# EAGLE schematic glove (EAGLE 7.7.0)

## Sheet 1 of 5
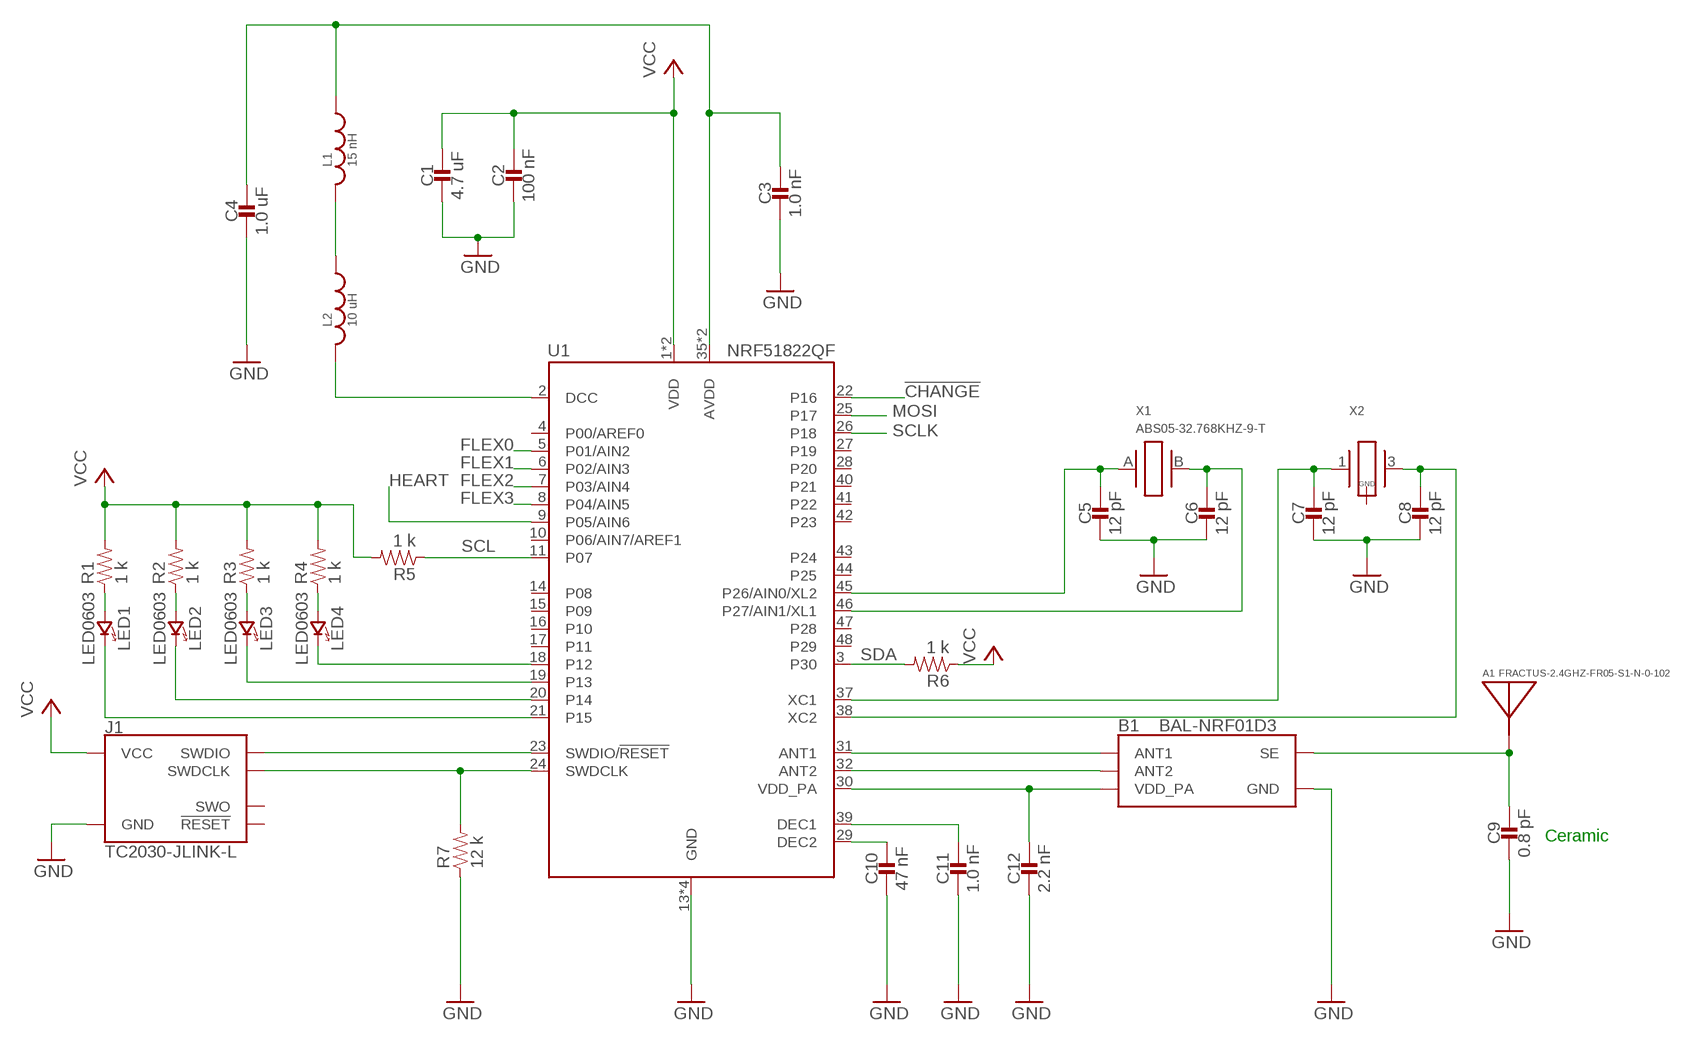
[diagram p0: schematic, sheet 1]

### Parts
A1  FRACTUS-2.4GHZ-FR05-S1-N-0-102  [FRACTUS-ANTENNA-FR05-S1-N-0-102]
B1  BAL-NRF01D3  [BAL-NRF01D3]
C1  4.7 uF  CAPACITOR0603_CAP  [0603_CAP]
C2  100 nF  CAPACITOR0402_CAP  [0402_CAP]
C3  1.0 nF  CAPACITOR0402_CAP  [0402_CAP]
C4  1.0 uF  CAPACITOR0603_CAP  [0603_CAP]
C5  12 pF  CAPACITOR0402_CAP  [0402_CAP]
C6  12 pF  CAPACITOR0402_CAP  [0402_CAP]
C7  12 pF  CAPACITOR0402_CAP  [0402_CAP]
C8  12 pF  CAPACITOR0402_CAP  [0402_CAP]
C9  0.8 pF  CAPACITOR0402_CAP  [0402_CAP]
C10  47 nF  CAPACITOR0402_CAP  [0402_CAP]
C11  1.0 nF  CAPACITOR0402_CAP  [0402_CAP]
C12  2.2 nF  CAPACITOR0402_CAP  [0402_CAP]
J1  TC2030-JLINK-L  [TC2030-IDC]
L1  15 nH  INDUCTOR0402  [0402_CAP]
L2  10 uH  INDUCTOR0603  [0603_CAP]
LED1  LED0603  [LED-0603]
LED2  LED0603  [LED-0603]
LED3  LED0603  [LED-0603]
LED4  LED0603  [LED-0603]
R1  1 k  RESISTOR0603_RES  [0603-RES]
R2  1 k  RESISTOR0603_RES  [0603-RES]
R3  1 k  RESISTOR0603_RES  [0603-RES]
R4  1 k  RESISTOR0603_RES  [0603-RES]
R5  1 k  RESISTOR0603_RES  [0603-RES]
R6  1 k  RESISTOR0603_RES  [0603-RES]
R7  12 k  RESISTOR0603_RES  [0603-RES]
U1  NRF51822QF  [QFN-48-6MM]
X1  ABS05-32.768KHZ-9-T  [ABS05]
X2  TXC-8Y  [TXC-8Y]

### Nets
!CHANGE: U1.22(P16) ; also sheet 3
FLEX0: U1.5(P01/AIN2) ; also sheet 5
FLEX1: U1.6(P02/AIN3) ; also sheet 5
FLEX2: U1.7(P03/AIN4) ; also sheet 5
FLEX3: U1.8(P04/AIN5) ; also sheet 5
GND: B1.GND C1.2 C2.2 C3.2 C4.2 C5.2 C6.2 C7.2 C8.2 C9.2 C10.2 C11.2 C12.2 J1.5(GND) R7.1 U1.13(GND) U1.33(GND) U1.34(GND) U1.GND ; also sheet 2,3,4,5
HEART: U1.9(P05/AIN6) ; also sheet 5
MOSI: U1.25(P17) ; also sheet 5
N$6: LED2.C(CATHODE) U1.20(P14)
N$8: LED2.A(ANODE) R2.1
N$10: LED1.C(CATHODE) U1.21(P15)
N$11: LED1.A(ANODE) R1.1
N$12: LED4.C(CATHODE) U1.18(P12)
N$13: LED4.A(ANODE) R4.1
N$14: L2.2 U1.2(DCC)
N$15: L1.2 L2.1
N$16: C3.1 C4.1 L1.1 U1.35(AVDD) U1.36(AVDD)
N$19: J1.2(SWDIO) U1.23(SWDIO/!RESET)
N$20: C8.1 U1.38(XC2) X2.3
N$21: B1.ANT1 U1.31(ANT1)
N$22: B1.ANT2 U1.32(ANT2)
N$23: B1.VCC(VDD_PA) C12.1 U1.30(VDD_PA)
N$24: A1.1(ANTENNA) B1.SE C9.1
N$25: C10.1 U1.29(DEC2)
N$26: C11.1 U1.39(DEC1)
N$27: C5.1 U1.45(P26/AIN0/XL2) X1.A
N$28: C6.1 U1.46(P27/AIN1/XL1) X1.B
N$29: C7.1 U1.37(XC1) X2.1
N$30: J1.4(SWDCLK) R7.2 U1.24(SWDCLK)
N$42: LED3.A(ANODE) R3.1
N$43: LED3.C(CATHODE) U1.19(P13)
SCL: R5.1 U1.11(P07) ; also sheet 2,3
SCLK: U1.26(P18) ; also sheet 5
SDA: R6.2 U1.3(P30) ; also sheet 2,3
VCC: C1.1 C2.1 J1.1(VCC) R1.2 R2.2 R3.2 R4.2 R5.2 R6.1 U1.1(VDD) U1.12(VDD) ; also sheet 2,3,4,5
Unconnected: J1.3(!RESET) J1.6(SWO) U1.4(P00/AREF0) U1.10(P06/AIN7/AREF1) U1.14(P08) U1.15(P09) U1.16(P10) U1.17(P11) U1.27(P19) U1.28(P20) U1.40(P21) U1.41(P22) U1.42(P23) U1.43(P24) U1.44(P25) U1.47(P28) U1.48(P29) X2.2(GND) X2.4(GND)

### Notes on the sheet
- Ceramic

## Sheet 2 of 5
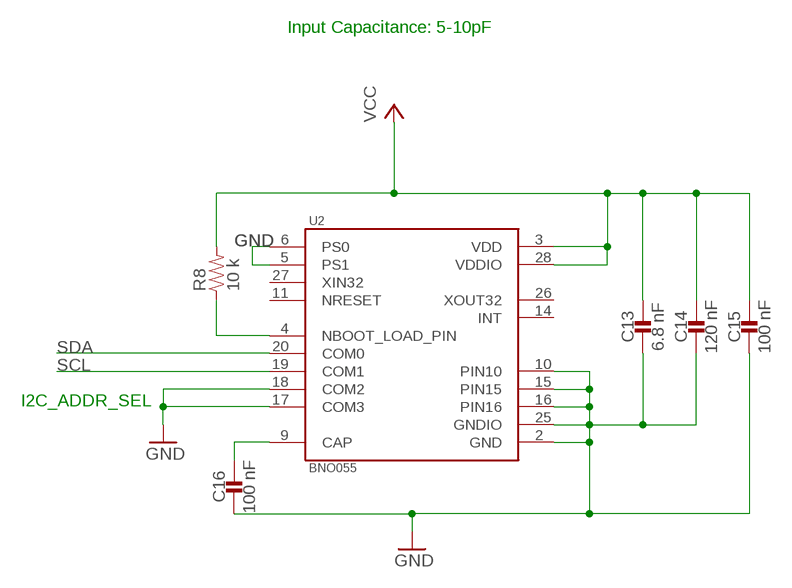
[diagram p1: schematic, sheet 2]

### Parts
C13  6.8 nF  CAPACITOR0603_CAP  [0603_CAP]
C14  120 nF  CAPACITOR0603_CAP  [0603_CAP]
C15  100 nF  CAPACITOR0603_CAP  [0603_CAP]
C16  100 nF  CAPACITOR0603_CAP  [0603_CAP]
R8  10 k  RESISTOR0603_RES  [0603-RES]
U2  BNO055  [LGA28R50P4X10_380X520X100]

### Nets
GND: C13.2 C14.2 C15.2 C16.2 U2.2(GND) U2.5(PS1) U2.6(PS0) U2.10(PIN10) U2.15(PIN15) U2.16(PIN16) U2.17(COM3) U2.18(COM2) U2.25(GNDIO) ; also sheet 1,3,4,5
N$9: C16.1 U2.9(CAP)
N$18: R8.1 U2.4(NBOOT_LOAD_PIN)
SCL: U2.19(COM1) ; also sheet 1,3
SDA: U2.20(COM0) ; also sheet 1,3
VCC: C13.1 C14.1 C15.1 R8.2 U2.3(VDD) U2.28(VDDIO) ; also sheet 1,3,4,5
Unconnected: U2.11(NRESET) U2.14(INT) U2.26(XOUT32) U2.27(XIN32)

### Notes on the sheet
- Input Capacitance: 5-10pF
- I2C_ADDR_SEL

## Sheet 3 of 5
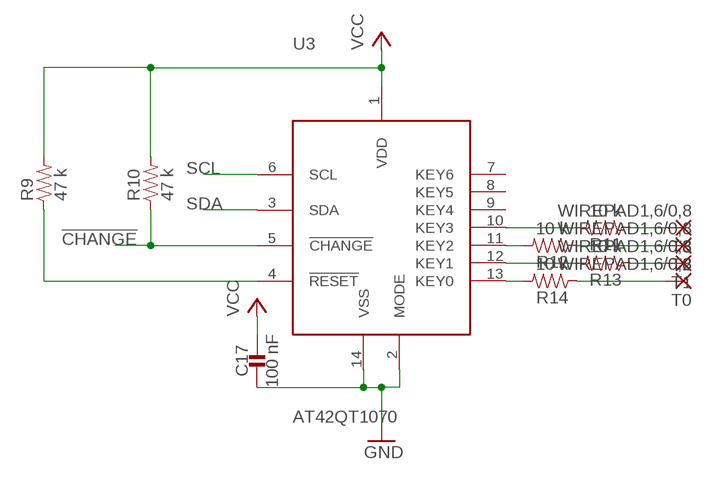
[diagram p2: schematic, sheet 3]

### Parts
C17  100 nF  CAPACITOR0603_CAP  [0603_CAP]
R9  47 k  RESISTOR0603_RES  [0603-RES]
R10  47 k  RESISTOR0603_RES  [0603-RES]
R11  10 k  RESISTOR0603_RES  [0603-RES]
R12  10 k  RESISTOR0603_RES  [0603-RES]
R13  10 k  RESISTOR0603_RES  [0603-RES]
R14  10 k  RESISTOR0603_RES  [0603-RES]
T0  WIREPAD1,6/0,8  [1,6/0,8]
T1  WIREPAD1,6/0,8  [1,6/0,8]
T2  WIREPAD1,6/0,8  [1,6/0,8]
T3  WIREPAD1,6/0,8  [1,6/0,8]
U3  AT42QT1070  [QT1070]

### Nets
!CHANGE: R10.1 U3.5(!CHANGE) ; also sheet 1
GND: C17.2 U3.2(MODE) U3.14(VSS) ; also sheet 1,2,4,5
N$31: R11.2 U3.10(KEY3)
N$32: R11.1 T3.1(P)
N$33: R12.2 U3.11(KEY2)
N$34: R12.1 T2.1(P)
N$35: R13.2 U3.12(KEY1)
N$36: R13.1 T1.1(P)
N$37: R14.2 U3.13(KEY0)
N$39: R14.1 T0.1(P)
N$40: R9.1 U3.4(!RESET)
SCL: U3.6(SCL) ; also sheet 1,2
SDA: U3.3(SDA) ; also sheet 1,2
VCC: C17.1 R9.2 R10.2 U3.1(VDD) ; also sheet 1,2,4,5
Unconnected: U3.7(KEY6) U3.8(KEY5) U3.9(KEY4)

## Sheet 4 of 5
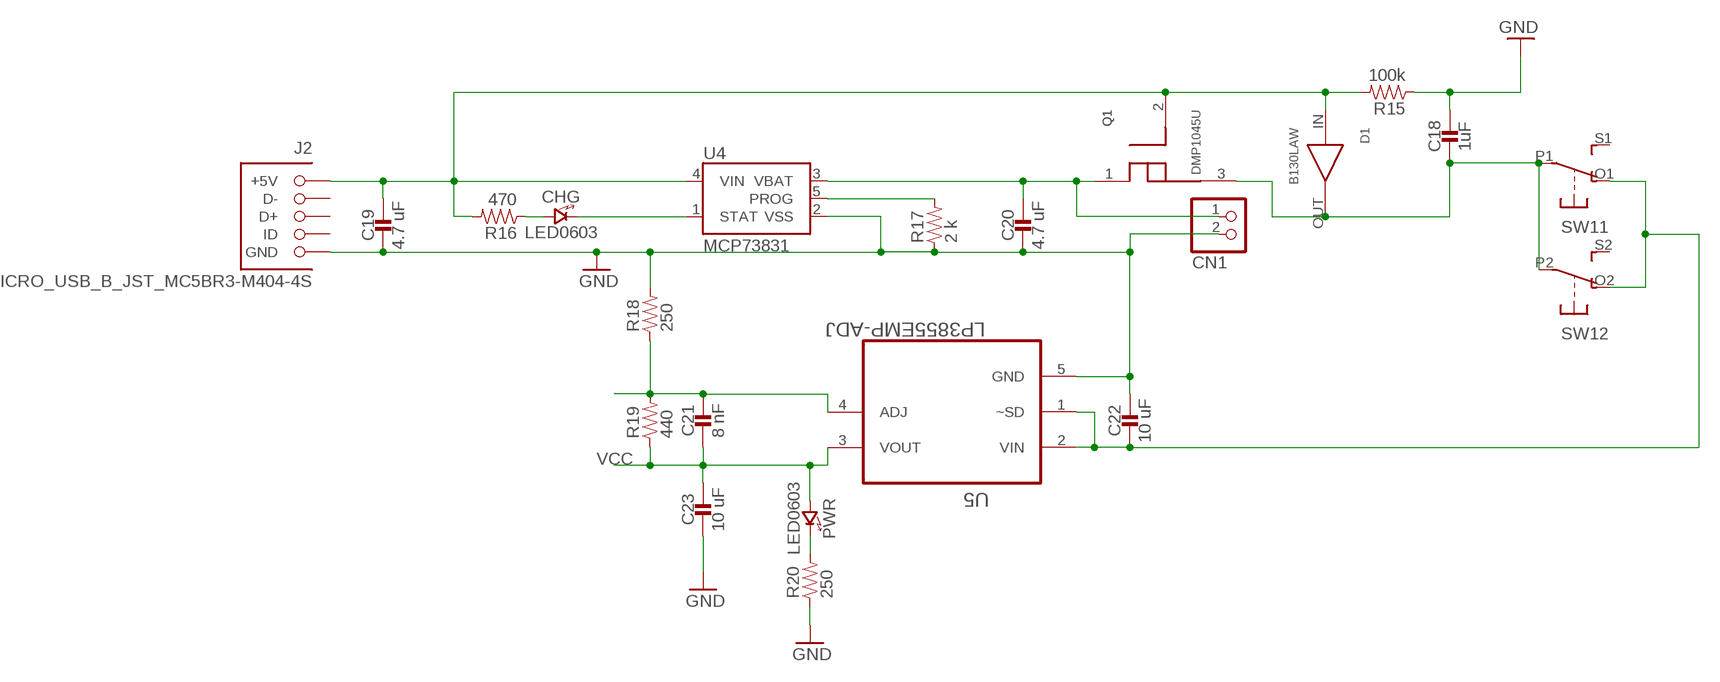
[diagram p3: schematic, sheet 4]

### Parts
C18  1uF  CAPACITOR0603_CAP  [0603_CAP]
C19  4.7 uF  CAPACITOR0603_CAP  [0603_CAP]
C20  4.7 uF  CAPACITOR0603_CAP  [0603_CAP]
C21  8 nF  CAPACITOR0603_CAP  [0603_CAP]
C22  10 uF  CAPACITOR0603_CAP  [0603_CAP]
C23  10 uF  CAPACITOR0603_CAP  [0603_CAP]
CHG  LED0603  [LED-0603]
CN1  JST_2PIN-SMT-RA  [JST-PH-2-SMT-RA]
D1  B130LAW  [2PIN]
J2  MICRO_USB_B_JST_MC5BR3-M404-4S  [USB_MICRO_B-JST-MC5BR3-M404-4S-TB]
PWR  LED0603  [LED-0603]
Q1  DMP1045U  [3PIN]
R15  100k  RESISTOR0603_RES  [0603-RES]
R16  470  RESISTOR0603_RES  [0603-RES]
R17  2 k  RESISTOR0603_RES  [0603-RES]
R18  250  RESISTOR0603_RES  [0603-RES]
R19  440  RESISTOR0603_RES  [0603-RES]
R20  250  RESISTOR0603_RES  [0603-RES]
SW1  DPDT-EG1390  [EG1390]
U4  MCP73831  [SOT23-5]
U5  LP3855EMP-ADJ  [SOT150P696X180-5N]

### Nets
GND: C18.1 C19.2 C20.2 C22.1 C23.2 CN1.2 J2.5(GND) R15.1 R17.1 R18.2 R20.1 U4.2(VSS) U5.5(GND) ; also sheet 1,2,3,5
N$1: C18.2 D1.OUT Q1.3(SOURCE) SW1.P1(1:P) SW1.P2(2:P)
N$2: CHG.A(ANODE) R16.1
N$3: CHG.C(CATHODE) U4.1(STAT)
N$4: R17.2 U4.5(PROG)
N$7: C21.1 R18.1 R19.2 U5.4(ADJ)
N$17: PWR.C(CATHODE) R20.2
N$38: C19.1 D1.IN J2.1(+5V) Q1.2(GATE) R15.2 R16.2 U4.4(VIN)
N$41: C20.1 CN1.1 Q1.1(DRAIN) U4.3(VBAT)
N$54: C22.2 SW1.O1(1:O) SW1.O2(2:O) U5.1(~SD) U5.2(VIN)
VCC: C21.2 C23.1 PWR.A(ANODE) R19.1 U5.3(VOUT) ; also sheet 1,2,3,5
Unconnected: J2.2(D-) J2.3(D+) J2.4(ID) SW1.S1(1:S) SW1.S2(2:S)

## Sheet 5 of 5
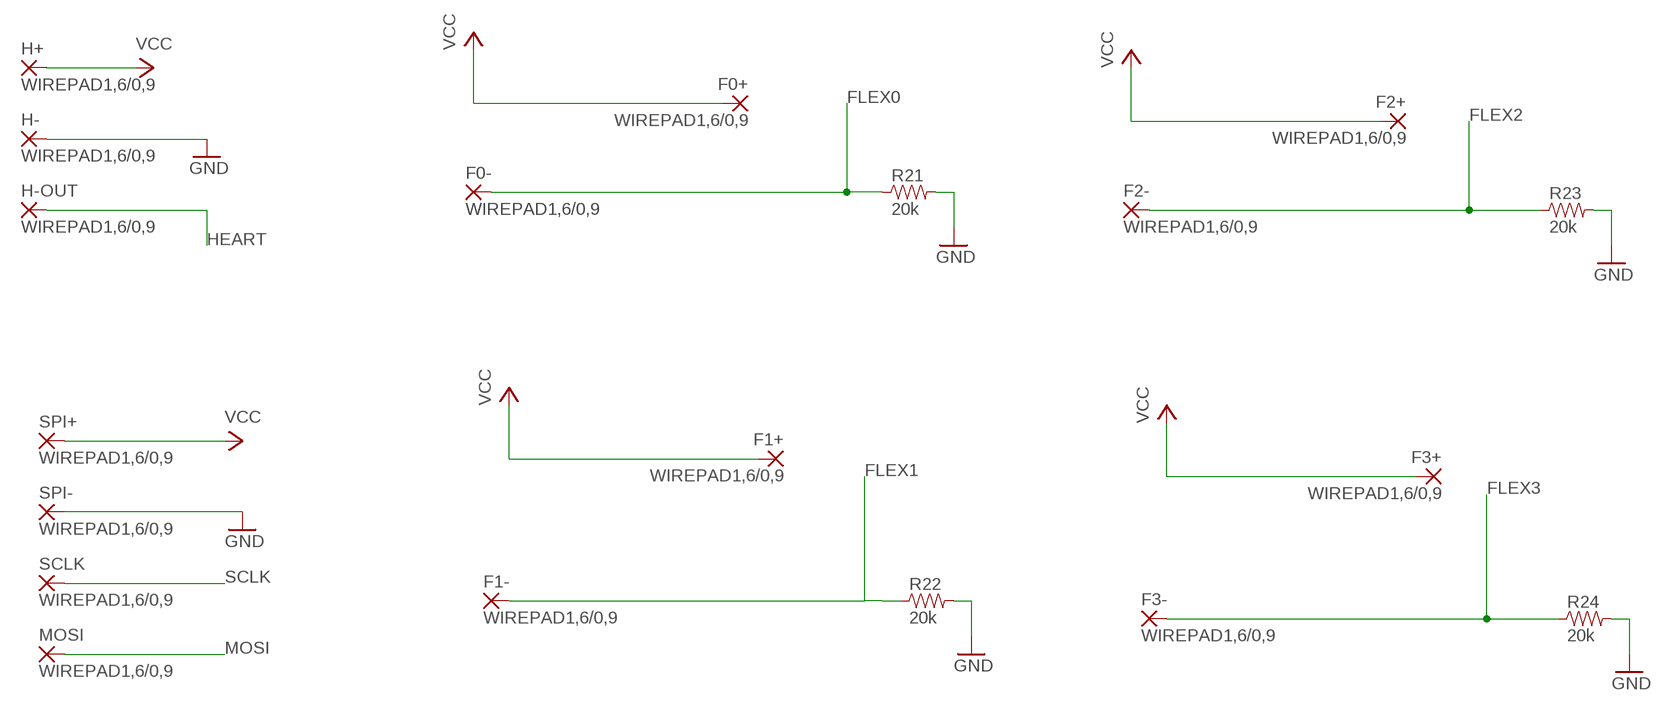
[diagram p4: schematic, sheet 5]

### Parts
F0+  WIREPAD1,6/0,9  [1,6/0,9]
F0-  WIREPAD1,6/0,9  [1,6/0,9]
F1+  WIREPAD1,6/0,9  [1,6/0,9]
F1-  WIREPAD1,6/0,9  [1,6/0,9]
F2+  WIREPAD1,6/0,9  [1,6/0,9]
F2-  WIREPAD1,6/0,9  [1,6/0,9]
F3+  WIREPAD1,6/0,9  [1,6/0,9]
F3-  WIREPAD1,6/0,9  [1,6/0,9]
H+  WIREPAD1,6/0,9  [1,6/0,9]
H-  WIREPAD1,6/0,9  [1,6/0,9]
H-OUT  WIREPAD1,6/0,9  [1,6/0,9]
MOSI  WIREPAD1,6/0,9  [1,6/0,9]
R21  20k  RESISTOR0603_RES  [0603-RES]
R22  20k  RESISTOR0603_RES  [0603-RES]
R23  20k  RESISTOR0603_RES  [0603-RES]
R24  20k  RESISTOR0603_RES  [0603-RES]
SCLK  WIREPAD1,6/0,9  [1,6/0,9]
SPI+  WIREPAD1,6/0,9  [1,6/0,9]
SPI-  WIREPAD1,6/0,9  [1,6/0,9]

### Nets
FLEX0: F0-.1(P) R21.1 ; also sheet 1
FLEX1: F1-.1(P) R22.1 ; also sheet 1
FLEX2: F2-.1(P) R23.1 ; also sheet 1
FLEX3: F3-.1(P) R24.1 ; also sheet 1
GND: H-.1(P) R21.2 R22.2 R23.2 R24.2 SPI-.1(P) ; also sheet 1,2,3,4
HEART: H-OUT.1(P) ; also sheet 1
MOSI: MOSI.1(P) ; also sheet 1
SCLK: SCLK.1(P) ; also sheet 1
VCC: F0+.1(P) F1+.1(P) F2+.1(P) F3+.1(P) H+.1(P) SPI+.1(P) ; also sheet 1,2,3,4

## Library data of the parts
A1 = chips:FRACTUS-2.4GHZ-FR05-S1-N-0-102: Fractus Compact Reach XtendTM chip antenna is engineered specifically for Bluetooth,; RICHARDSON_RFPD: FR05-S1-N-0102B
B1 = chips:BAL-NRF01D3: 50 ohm nominal input / conjugate match balun to nRF51422-QFAA, nRF24LE1, nRF51822-QFAA/AB, with integrated harmonic filter; DIGIKEY: 497-13637-1-ND; MOUSER: 511-BAL-NRF01D3
C1-C23 = passives:CAPACITOR: 0402 Capacitor
CHG LED1-LED4 PWR = leds:LED: LED
CN1 = adafruit:JST_2PIN: JST 2-Pin Connectors of various flavors
D1 = load_balance:B130LAW
F0+ F0- F1+ F1- F2+ F2- F3+ F3- H+ H- H-OUT MOSI SCLK SPI+ SPI- T0 T1-T3 = wirepad:WIREPAD: Wire PAD connect wire on PCB
J1 = connector:TC2030-JLINK
J2 = connector:MICRO_USB_B_JST_MC5BR3-M404-4S: Micro USB B mid mount; DIGIKEY: 455-2567-2-ND; MOUSER: 53X3655
L1 L2 = passives:INDUCTOR: A very specific inductor
Q1 = load_balance:DMP1045U
R1-R24 = passives:RESISTOR: Resistor
SW1 = adafruit:DPDT
U1 = chips:NRF51822: Multiprotocol Bluetooth� 4.0 low energy/2.4 GHz RF SoC; DIGIKEY: 1490-1032-1-ND; MOUSER: 949-NRF51822-QFAB-R7
U2 = BNO055:BNO055: BNO055 9-axis Absolute Orientation Sensor ( SiP ) w/Sensors and Sensor Fusion; AVAILABILITY: Good; DESCRIPTION: BNO055 9-axis Absolute Orientation Sensor ( SiP ) w/Sensors and Sensor Fusion; MF: Bosch; MP: BNO055; PACKAGE: LGA-28 Bosch; PRICE: 9.48 USD
U3 = QT1070:AT42QT1070
U4 = SparkFun-PowerIC:MCP73831: Miniature single cell, fully integrated Li-Ion, Li-polymer charge management controller http://ww1.microchip.com/downloads/en/DeviceDoc/21984a.pdf
U5 = LP3855EMP-ADJ:LP3855EMP-ADJ: Linear Regulators; AVAILABILITY: Good; DESCRIPTION: 1.5A Fast Response Ultra Low Dropout Linear Regulators 5-SOT-223 -40 to 125; MF: Texas Instruments; MP: LP3855EMP-ADJ; PACKAGE: SOT-223 Texas Instruments; PRICE: 3.03 USD
X1 = crystals:ABS05-32.768KHZ: 32.768kHz Crystal; DIGIKEY: 535-11897-1-ND
X2 = crystals:TXC-8Y: 2mmx1.6mm SMD Crystal

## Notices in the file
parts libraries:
SparkFun-PowerIC: Licensing: CC v3.0 Share-Alike You are welcome to use this library for commercial purposes.
